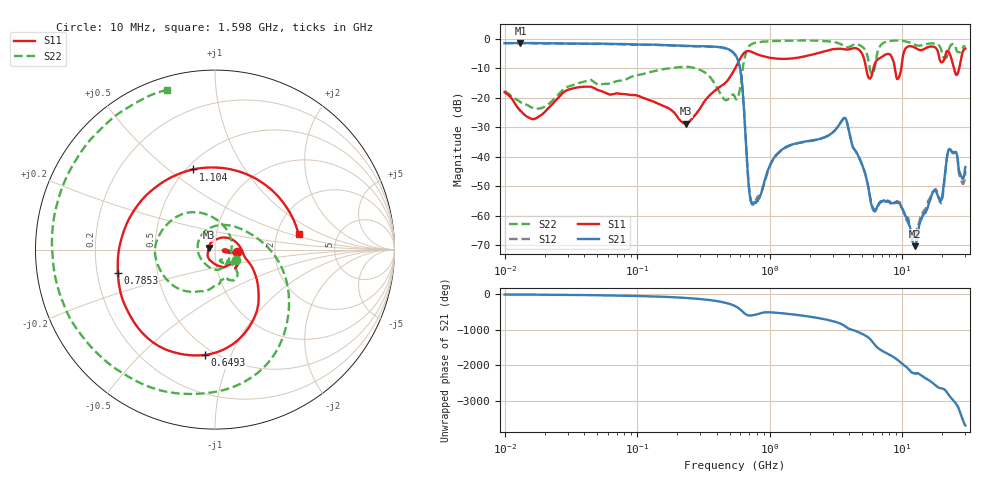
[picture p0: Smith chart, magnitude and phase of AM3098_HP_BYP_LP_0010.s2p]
!Agilent Technologies,E8364B,MY43040894,A.07.50.67
!Agilent E8364B: A.07.50.67
!Date: Wednesday, June 17, 2020 09:19:42
!Correction: S11(Full 2 Port(1,2))
!S21(Full 2 Port(1,2))
!S12(Full 2 Port(1,2))
!S22(Full 2 Port(1,2))
!S2P File: Measurements: S11, S21, S12, S22:Log Frequency Sweep
# Hz S  dB  R 50
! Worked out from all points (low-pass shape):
!   1601 points, 10 MHz to 30 GHz, reference 50 ohm
!   highest |S21| = -1.41 dB at 13.17 MHz (marker M1); lowest = -70.4 dB at 12.5 GHz (marker M2)
!   |S21| within 3 dB of the highest: start of sweep to 524.1 MHz
!   lowest |S11| = -28.8 dB at 233.9 MHz (marker M3), VSWR 1.08, Z = 46.6 + j1.01 ohm
!   |S11| at or under -10 dB: 5.344 GHz to 6.072 GHz (727.5 MHz wide, 12.7 % of centre); 8.811 GHz to 9.848 GHz (1.036 GHz wide, 11.1 % of centre); 24.61 GHz to 26.94 GHz (2.336 GHz wide, 9.06 % of centre)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
!   |S22| runs from -23.8 to -0.6 dB; largest |S21 - S12| = 0.015
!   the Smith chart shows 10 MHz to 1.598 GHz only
!   S11 on the Smith chart (normalised r, x): 10 MHz: 1.28, -0.03; 649.3 MHz: 0.45, -0.80; 785.3 MHz: 0.29, -0.11; 1.104 GHz: 0.54, +0.61; 1.598 GHz: 2.64, +0.60
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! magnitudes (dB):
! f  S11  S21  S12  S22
! 10 MHz  -18.1  -1.5  -1.5  -17.7
! 13.17 MHz  -24.5  -1.4  -1.5  -21.5
! 38.04 MHz  -16.3  -1.7  -1.7  -14.8
! 144.7 MHz  -22.0  -2.1  -2.1  -10.6
! 233.9 MHz  -28.8  -2.4  -2.5  -9.5
! 547.7 MHz  -10.1  -5.3  -5.4  -19.8
! 602.4 MHz  -6.6  -10.8  -10.9  -16.1
! 649.3 MHz  -4.6  -28.5  -28.5  -6.3
! 710.5 MHz  -4.2  -53.7  -53.2  -2.2
! 785.3 MHz  -5.1  -55.5  -54.9  -1.4
! 1.104 GHz  -6.7  -39.8  -40.0  -0.8
! 1.598 GHz  -6.5  -35.5  -35.5  -0.6
! 2.084 GHz  -5.4  -34.5  -34.6  -0.6
! 3.704 GHz  -3.6  -26.9  -27.0  -2.6
! 6.019 GHz  -10.8  -57.8  -57.4  -11.7
! 7.926 GHz  -5.2  -55.3  -55.1  -0.8
! 9.302 GHz  -13.6  -55.5  -55.2  -0.6
! 12.5 GHz  -3.0  -70.4  -67.2  -2.0
! 19.8 GHz  -8.0  -54.6  -55.5  -4.0
! 22.67 GHz  -4.8  -37.4  -37.7  -3.3
! 25.82 GHz  -12.3  -39.2  -39.4  -4.1
! 30 GHz  -3.3  -43.5  -44.8  -2.6
